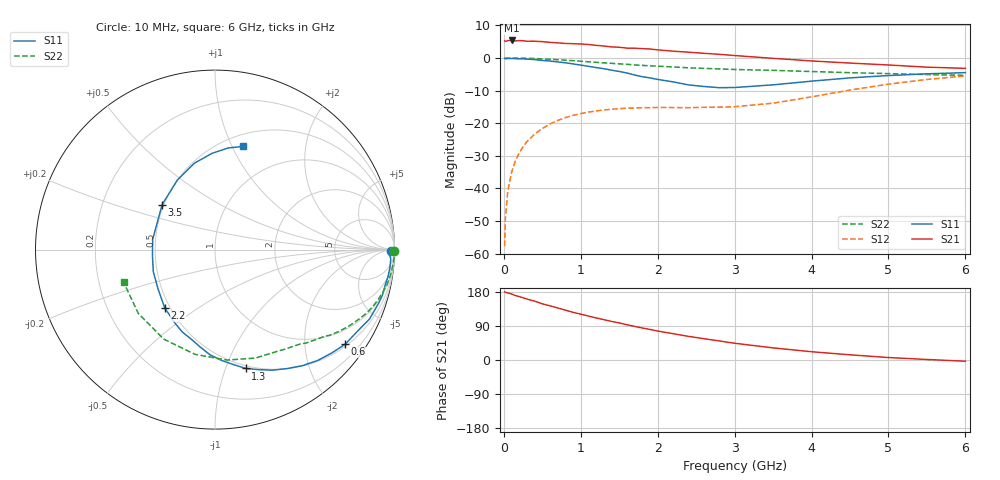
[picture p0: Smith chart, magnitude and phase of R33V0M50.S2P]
! SIEMENS Small Signal Semiconductors
! BFR181
! Si NPN RF Bipolar Junction Transistor in SOT23
! VCE = 3 V  IC = 0.5 mA
! Common Emitter S-Parameters:  May  1996
# GHz  S  MA  R  50
!  f  S11  S21  S12  S22
! GHz  MAG  ANG  MAG  ANG  MAG  ANG  MAG  ANG
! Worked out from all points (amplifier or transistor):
!   36 points, 10 MHz to 6 GHz, reference 50 ohm
!   highest |S21| = 5.4 dB at 100 MHz (marker M1)
!   |S21| within 3 dB of that: start of sweep to 2.059 GHz
!   unconditionally stable (mu >= 1): 2.354 GHz to 3.957 GHz
!   at 250 MHz: K = 0.12, MSG = 16.3 dB, |S12| = -27.3 dB
!   at 1.4 GHz: K = 0.61, MSG = 9.6 dB, |S12| = -15.7 dB
!   at 6 GHz: K = 0.92, MSG = 1.2 dB, |S12| = -5.5 dB
!   S11 on the Smith chart (normalised r, x): 10 MHz: 85, -37; 600 MHz: 0.55, -2.98; 1.3 GHz: 0.47, -1.18; 2.2 GHz: 0.47, -0.37; 3.5 GHz: 0.49, +0.29; 6 GHz: 0.62, +1.10
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0.01  0.9804 -0.5  1.833 179.8  0.0013 93.3  0.9997 -0.3
0.02  0.97 -1.2  1.789 178.6  0.0035 92.1  0.9886 -0.6
0.05  0.9808 -3.0  1.842 177.0  0.0088 89.3  0.9978 -1.4
0.1  0.9797 -6.0  1.853 174.2  0.0176 85.5  0.9988 -2.8
0.15  0.9755 -8.9  1.82 170.1  0.0265 82.6  0.9958 -4.4
0.2  0.9683 -11.8  1.846 167.3  0.0349 81.3  0.9931 -5.7
0.3  0.9595 -18.1  1.801 160.8  0.0519 77.4  0.9865 -8.6
0.4  0.9438 -24.2  1.805 155.4  0.0679 73.3  0.9791 -11.3
0.5  0.9134 -30.2  1.777 148.2  0.0826 69.5  0.9657 -14.0
0.6  0.8967 -36.0  1.733 143.0  0.0972 65.5  0.953 -16.6
0.9  0.8097 -53.0  1.653 125.8  0.1317 55.0  0.9078 -23.7
1.1  0.7442 -64.5  1.606 115.9  0.1477 49.1  0.8726 -28.0
1.3  0.6839 -75.5  1.522 106.5  0.1594 44.1  0.8407 -31.8
1.8  0.5153 -105.1  1.388 84.4  0.1728 36.2  0.7684 -39.6
2.2  0.4296 -130.6  1.269 69.4  0.1736 33.5  0.7275 -45.6
2.4  0.386 -145.2  1.225 62.4  0.1725 34.5  0.7054 -48.5
2.8  0.3499 -175.1  1.136 50.3  0.1759 37.7  0.6785 -54.8
3.5  0.3867 139.6  0.986 32.0  0.2025 46.9  0.645 -69.5
4.5  0.4947 103.5  0.834 13.7  0.3217 49.9  0.5941 -100.8
5  0.5368 91.7  0.78 6.5  0.3964 44.8  0.5747 -119.8
5.5  0.5707 82.7  0.722 1.4  0.4671 37.3  0.556 -140.2
6  0.595 75.0  0.692 -3.2  0.5295 28.5  0.5405 -160.3
